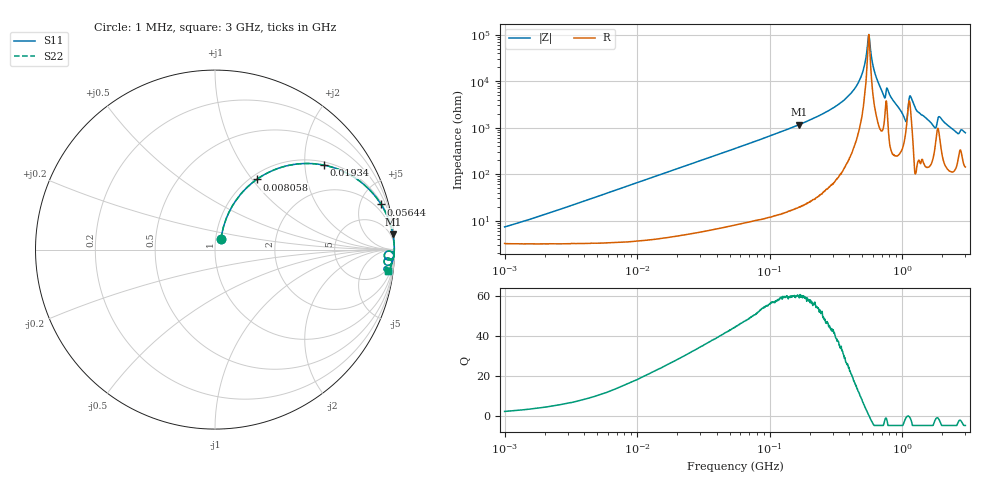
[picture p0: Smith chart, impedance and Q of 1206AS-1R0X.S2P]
!s-Parameter Generated by FASTRON Sdn. Bhd.
!FASTRON P/N : 1206AS-1R0X
!Keysight Technologies: E4991B_MY54100416_A.01.15
!Date created: Thu Nov 16 13:38:19 2023
!Version  : Rev00 Thu Nov 16 13:38:19 2023
!Data & Calibration Information:
!Freq	S11	S21	S12	S22
!PortZ  Port1:50+j0  Port2:50+j0
!When reading reference impedance value at option line is always used.
! Remarks : This data is being provided solely for informational purposes.
# Hz S dB R 50
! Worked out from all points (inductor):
!   1601 points, 1 MHz to 3 GHz, reference 50 ohm
!   read as one part in series: L = 1.04 uH near 1.441 MHz
!   highest Q = 60.2 at 166.3 MHz (marker M1), where L = 1.11 uH
!   self-resonance near 558.4 MHz
!   S11 on the Smith chart (normalised r, x): 1 MHz: 1.06, +0.13; 8.058 MHz: 1.07, +1.05; 19.34 MHz: 1.09, +2.51; 56.44 MHz: 1.16, +7.32; 3 GHz: 4, -15
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1000000  -23.03 60.3  -0.29 -3.6  -0.29 -3.6  -23.03 60.3
3804036  -12.53 69.1  -0.52 -13.6  -0.52 -13.6  -12.53 69.1
8057953  -6.85 59.3  -1.29 -27.0  -1.29 -27.0  -6.85 59.3
1.447069e7  -3.46 45.4  -2.94 -42.2  -2.94 -42.2  -3.46 45.4
1.934349e7  -2.28 37.7  -4.27 -50.2  -4.27 -50.2  -2.28 37.7
5.477226e7  -0.38 15.6  -11.39 -73.1  -11.39 -73.1  -0.38 15.6
5.644167e7  -0.36 15.2  -11.63 -73.5  -11.63 -73.5  -0.36 15.2
1.663456e8  -0.04 4.9  -21.31 -84.1  -21.31 -84.1  -0.04 4.9
2.083556e8  -0.03 3.7  -23.72 -85.3  -23.72 -85.3  -0.03 3.7
4.282981e8  -0.01 0.9  -36.06 -85.9  -36.06 -85.9  -0.01 0.9
4.976708e8  -0.01 0.4  -43.04 -82.4  -43.04 -82.4  -0.01 0.4
5.583748e8  -0.01 0.0  -59.69 -11.7  -59.69 -11.7  -0.01 0.0
6.685918e8  -0.01 -0.7  -38.64 82.1  -38.64 82.1  -0.01 -0.7
7.207075e8  -0.03 -1.1  -34.34 78.1  -34.34 78.1  -0.03 -1.1
7.925923e8  -0.02 -1.0  -35.13 82.2  -35.13 82.2  -0.02 -1.0
1.048936e9  -0.25 -3.4  -23.73 62.9  -23.73 62.9  -0.25 -3.4
1.165162e9  -0.08 -1.1  -33.22 64.0  -33.22 64.0  -0.08 -1.1
1.307284e9  -0.04 -2.6  -26.94 82.8  -26.94 82.8  -0.04 -2.6
1.730092e9  -0.23 -5.1  -20.78 71.2  -20.78 71.2  -0.23 -5.1
1.931433e9  -0.17 -3.2  -24.67 68.7  -24.67 68.7  -0.17 -3.2
2.568929e9  -0.26 -7.0  -18.18 72.5  -18.18 72.5  -0.26 -7.0
3e9  -0.27 -7.1  -18.06 72.4  -18.06 72.4  -0.27 -7.1
